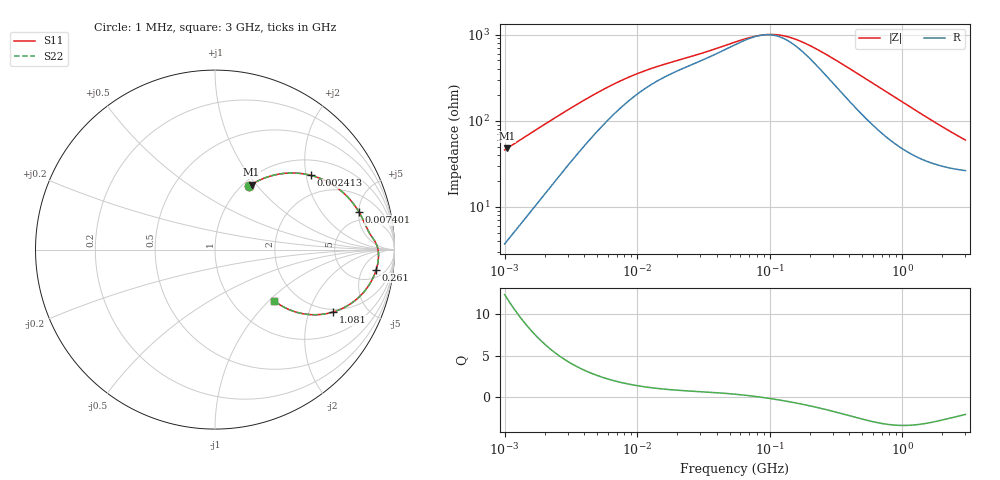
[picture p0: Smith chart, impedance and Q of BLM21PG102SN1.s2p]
! BLM21PG102SN1
# Hz S RI R 50
!Freq.(Hz) S11(Real) S11(Imag) S21(Real) S21(Imag) S12(Real) S12(Imag) S22(Real) S22(Imag)
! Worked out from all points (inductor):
!   401 points, 1 MHz to 3 GHz, reference 50 ohm
!   read as one part in series: L = 7.21 uH near 1.041 MHz
!   highest Q = 11.9 at 1.041 MHz (marker M1), where L = 7.24 uH
!   self-resonance near 88.87 MHz
!   S11 on the Smith chart (normalised r, x): 1 MHz: 1.07, +0.91; 2.413 MHz: 1.40, +2.13; 7.401 MHz: 3.76, +5.04; 261 MHz: 8, -10; 1.081 GHz: 1.88, -2.93; 3 GHz: 1.53, -1.07
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1000000  0.1913 0.3548  0.8087 -0.3548  0.8087 -0.3548  0.1913 0.3548
1040844  0.2034 0.3626  0.7966 -0.3626  0.7966 -0.3626  0.2034 0.3626
1616692  0.3663 0.4224  0.6337 -0.4224  0.6337 -0.4224  0.3663 0.4224
1974946  0.451 0.4263  0.549 -0.4263  0.549 -0.4263  0.451 0.4263
2412589  0.5338 0.4137  0.4662 -0.4137  0.4662 -0.4137  0.5338 0.4137
3823119  0.6882 0.3388  0.3118 -0.3388  0.3118 -0.3388  0.6882 0.3388
5266264  0.757 0.2732  0.243 -0.2732  0.243 -0.2732  0.757 0.2732
7400828  0.8017 0.2099  0.1983 -0.2099  0.1983 -0.2099  0.8017 0.2099
1.461624e7  0.8448 0.1228  0.1552 -0.1228  0.1552 -0.1228  0.8448 0.1228
5.477226e7  0.8962 0.0359  0.1038 -0.0359  0.1038 -0.0359  0.8962 0.0359
8.011685e7  0.9063 0.00824  0.0937 -0.00824  0.0937 -0.00824  0.9063 0.00824
1.081723e8  0.9104 -0.0165  0.0896 0.0165  0.0896 0.0165  0.9104 -0.0165
1.460522e8  0.9108 -0.0443  0.0892 0.0443  0.0892 0.0443  0.9108 -0.0443
2.094008e8  0.9056 -0.0834  0.0944 0.0834  0.0944 0.0834  0.9056 -0.0834
2.609752e8  0.8984 -0.1117  0.1016 0.1117  0.1016 0.1117  0.8984 -0.1117
4.853736e8  0.848 -0.2126  0.152 0.2126  0.152 0.2126  0.848 -0.2126
8.005644e8  0.7501 -0.3055  0.2499 0.3055  0.2499 0.3055  0.7501 -0.3055
1.080907e9  0.6591 -0.3475  0.3409 0.3475  0.3409 0.3475  0.6591 -0.3475
1.374365e9  0.5739 -0.3625  0.4261 0.3625  0.4261 0.3625  0.5739 -0.3625
1.712864e9  0.494 -0.358  0.506 0.358  0.506 0.358  0.494 -0.358
2.359433e9  0.3896 -0.3236  0.6104 0.3236  0.6104 0.3236  0.3896 -0.3236
3e9  0.328 -0.284  0.672 0.284  0.672 0.284  0.328 -0.284
